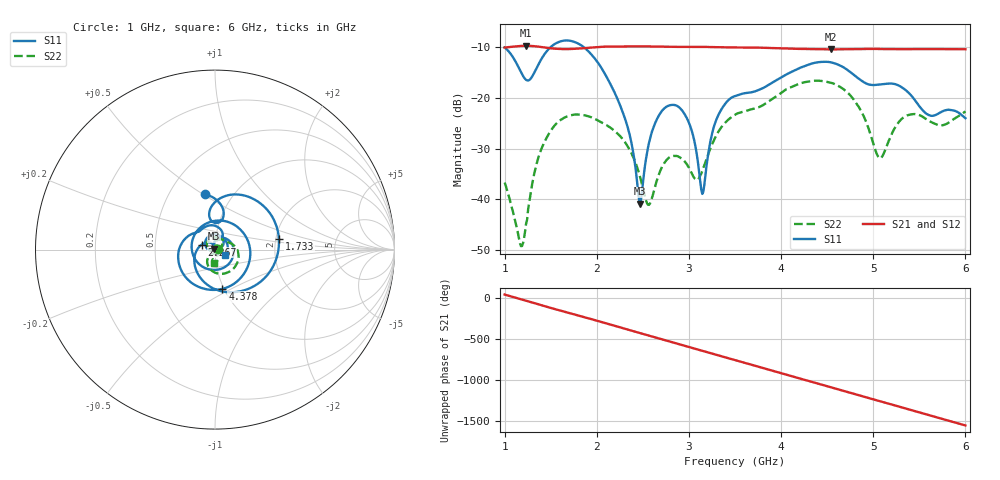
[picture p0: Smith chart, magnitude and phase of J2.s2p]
!Agilent Technologies,E8364B,MY43040528,A.07.50.67
!Agilent E8364B: A.07.50.67
!Date: Sunday, March 01, 2026 18:57:08
!Correction: S11(Full 2 Port(1,2))
!S21(Full 2 Port(1,2))
!S12(Full 2 Port(1,2))
!S22(Full 2 Port(1,2))
!S2P File: Measurements: S11, S21, S12, S22:
# Hz S  dB  R 50
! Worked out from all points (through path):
!   451 points, 1 GHz to 6 GHz, reference 50 ohm
!   highest |S21| = -9.74 dB at 1.233 GHz (marker M1); lowest = -10.5 dB at 4.544 GHz (marker M2)
!   group delay of S21, straight-line fit = 890 ps
!   lowest |S11| = -40.8 dB at 2.467 GHz (marker M3), VSWR 1.02, Z = 49.3 + j0.568 ohm
!   |S11| at or under -10 dB: start of sweep to 1.499 GHz; 1.858 GHz to end of sweep
!   |S22| runs from -49.2 to -16.6 dB; largest |S21 - S12| = 0.0015
!   S11 on the Smith chart (normalised r, x): 1 GHz: 0.74, +0.51; 1.733 GHz: 2.08, +0.29; 2.267 GHz: 0.86, +0.05; 4.378 GHz: 0.98, -0.45; 6 GHz: 1.12, -0.07
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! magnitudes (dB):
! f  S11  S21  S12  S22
! 1 GHz  -10.1  -10.1  -10.1  -36.7
! 1.178 GHz  -14.9  -9.8  -9.8  -49.2
! 1.233 GHz  -16.5  -9.7  -9.8  -44.8
! 1.411 GHz  -12.0  -10.0  -10.0  -29.5
! 1.733 GHz  -8.8  -10.4  -10.4  -23.4
! 1.844 GHz  -9.8  -10.2  -10.3  -23.4
! 2.267 GHz  -22.1  -9.9  -9.9  -27.8
! 2.467 GHz  -40.8  -9.8  -9.9  -35.3
! 2.567 GHz  -28.9  -9.9  -9.9  -41.1
! 2.667 GHz  -23.7  -9.9  -9.9  -35.5
! 2.956 GHz  -23.3  -10.0  -10.0  -32.5
! 3.144 GHz  -38.9  -10.0  -10.0  -34.4
! 3.289 GHz  -24.7  -10.0  -10.0  -27.7
! 3.5 GHz  -19.6  -10.1  -10.1  -23.3
! 4.344 GHz  -13.2  -10.4  -10.4  -16.7
! 4.378 GHz  -13.0  -10.4  -10.4  -16.6
! 4.544 GHz  -13.0  -10.5  -10.5  -17.0
! 4.833 GHz  -16.1  -10.4  -10.4  -21.5
! 5.056 GHz  -17.4  -10.4  -10.4  -31.6
! 5.167 GHz  -17.2  -10.4  -10.4  -28.5
! 5.378 GHz  -18.9  -10.4  -10.4  -23.4
! 6 GHz  -24.0  -10.4  -10.5  -22.6
